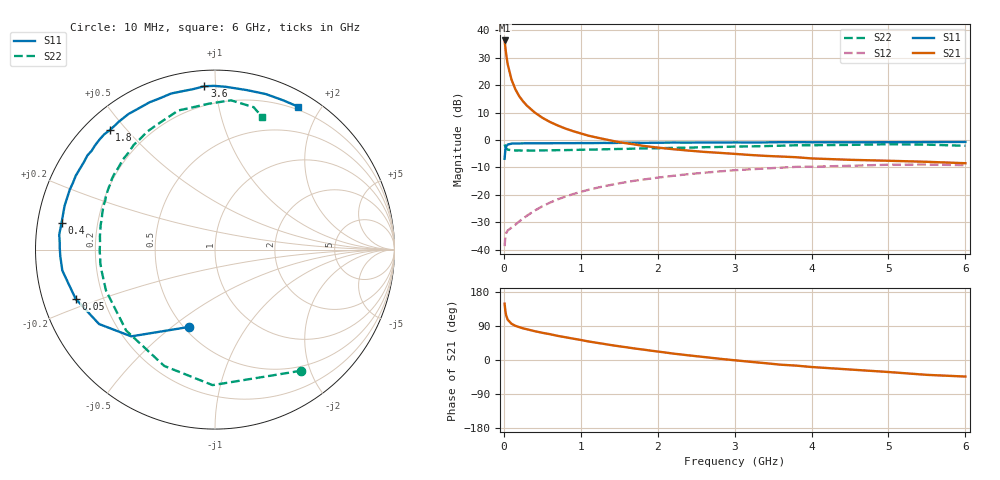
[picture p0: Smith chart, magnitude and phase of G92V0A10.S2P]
! SIEMENS Small Signal Semiconductors
! BFG235
! Si NPN RF Bipolar Junction Transistor in SOT223
! VCE = 2 V  IC = 100 mA
! Common Emitter S-Parameters:  July  1994
# GHz  S  MA  R  50
!  f  S11  S21  S12  S22
! GHz  MAG  ANG  MAG  ANG  MAG  ANG  MAG  ANG
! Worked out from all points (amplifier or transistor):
!   40 points, 10 MHz to 6 GHz, reference 50 ohm
!   highest |S21| = 36.3 dB at 10 MHz (marker M1)
!   |S21| within 3 dB of that: start of sweep to 21.93 MHz
!   unconditionally stable (mu >= 1): 454.9 MHz to 1.596 GHz; 1.79 GHz to 1.828 GHz
!   at 200 MHz: K = 0.79, MSG = 22.8 dB, |S12| = -29.7 dB
!   at 1.5 GHz: K = 1.01, MAG = 6.9 dB, |S12| = -15.8 dB
!   at 6 GHz: K = 0.93, MSG = 0.4 dB, |S12| = -9.2 dB
!   S11 on the Smith chart (normalised r, x): 10 MHz: 0.53, -0.58; 50 MHz: 0.10, -0.17; 400 MHz: 0.07, +0.09; 1.8 GHz: 0.07, +0.45; 3.6 GHz: 0.09, +0.93; 6 GHz: 0.16, +1.72
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0.01  0.4539 -108.4  65.12 148.6  0.0116 59.5  0.8287 -54.5
0.02  0.672 -134.0  48.6 129.0  0.0176 44.3  0.7552 -91.0
0.03  0.7677 -147.3  36.98 117.7  0.02 36.8  0.7072 -113.6
0.05  0.8236 -160.6  24.03 106.3  0.0224 31.1  0.6696 -137.7
0.1  0.8586 -172.2  12.54 95.6  0.0253 34.4  0.6487 -159.4
0.15  0.8626 -177.5  8.385 90.2  0.0286 40.3  0.6426 -168.2
0.2  0.8649 179.5  6.272 86.7  0.0328 45.3  0.6435 -173.1
0.25  0.8671 176.7  5.052 83.5  0.037 49.0  0.641 -176.5
0.3  0.872 174.5  4.222 81.1  0.0416 52.4  0.6427 -179.4
0.4  0.8678 170.2  3.18 76.1  0.0515 55.8  0.6414 176.7
0.5  0.8692 166.7  2.543 71.8  0.0618 57.5  0.6455 173.4
0.7  0.8732 160.1  1.839 63.7  0.0828 58.2  0.6521 167.7
0.9  0.8745 154.9  1.448 56.4  0.1032 56.1  0.6579 162.9
1.1  0.8772 148.5  1.197 48.9  0.1235 53.7  0.6677 158.1
1.4  0.8806 141.3  0.971 39.2  0.1524 48.9  0.6812 151.7
1.8  0.887 131.5  0.786 27.8  0.1888 41.8  0.701 143.5
2.2  0.8962 122.6  0.679 17.0  0.222 34.2  0.7178 135.5
3.2  0.9009 101.6  0.533 -4.7  0.2919 14.9  0.7636 116.6
3.6  0.9122 93.7  0.499 -12.4  0.3129 6.5  0.7863 108.3
4.5  0.9063 78.5  0.435 -25.1  0.3387 -9.2  0.8135 92.5
5.5  0.9143 65.5  0.4 -39.2  0.3573 -26.9  0.8221 74.8
6  0.921 59.9  0.377 -43.7  0.3468 -33.5  0.7833 70.3
